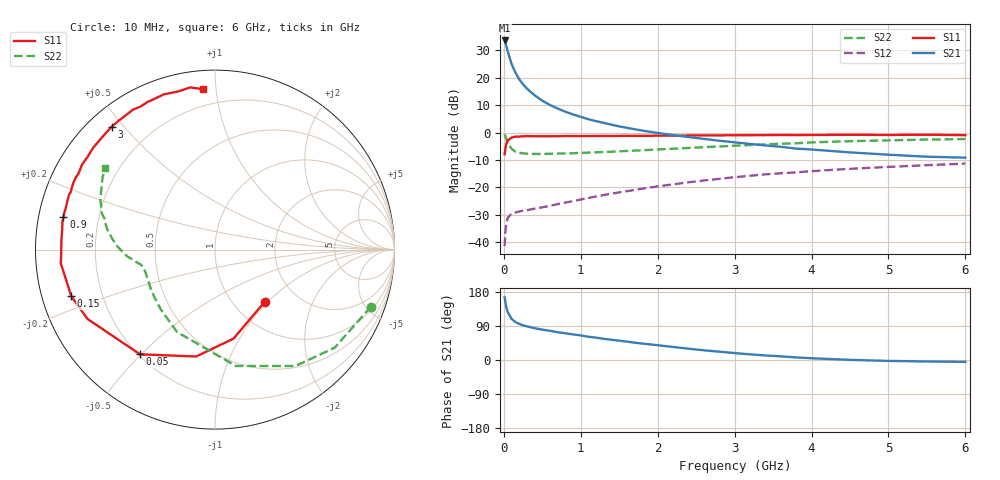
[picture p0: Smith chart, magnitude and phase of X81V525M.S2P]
! SIEMENS Small Signal Semiconductors
! BFP136W
! Si NPN RF Bipolar Junction Transistor in SOT343
! VCE = 1.5 V  IC = 25 mA
! Common Emitter S-Parameters:  September  1994
# GHz  S  MA  R  50
!  f  S11  S21  S12  S22
! GHz  MAG  ANG  MAG  ANG  MAG  ANG  MAG  ANG
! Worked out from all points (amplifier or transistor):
!   40 points, 10 MHz to 6 GHz, reference 50 ohm
!   highest |S21| = 33.6 dB at 10 MHz (marker M1)
!   |S21| within 3 dB of that: start of sweep to 41.63 MHz
!   unconditionally stable (mu >= 1): 768.6 MHz to 2.874 GHz
!   at 200 MHz: K = 0.39, MSG = 24.1 dB, |S12| = -28.8 dB
!   at 1.5 GHz: K = 1.16, MAG = 9.6 dB, |S12| = -21.8 dB
!   at 6 GHz: K = 1.00, MSG = 1.1 dB, |S12| = -11.3 dB
!   S11 on the Smith chart (normalised r, x): 10 MHz: 1.38, -0.96; 50 MHz: 0.21, -0.50; 150 MHz: 0.09, -0.16; 900 MHz: 0.07, +0.10; 3 GHz: 0.07, +0.46; 6 GHz: 0.10, +0.92
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0.01  0.4017 -46.4  47.72 165.4  0.0085 74.6  0.9248 -20.1
0.02  0.5068 -78.3  43.52 152.2  0.0155 63.8  0.8623 -39.3
0.03  0.6048 -100.0  39.22 141.5  0.0213 54.4  0.7888 -55.3
0.05  0.7175 -125.6  30.34 126.3  0.0278 41.0  0.659 -79.8
0.1  0.8089 -151.5  17.9 108.6  0.0334 28.8  0.5053 -114.8
0.15  0.842 -162.1  12.38 100.2  0.0349 25.6  0.4496 -132.3
0.2  0.8457 -167.9  9.362 95.2  0.0364 25.2  0.4282 -142.6
0.25  0.8538 -172.0  7.568 91.5  0.0376 26.1  0.4184 -149.1
0.3  0.8624 -174.8  6.342 88.8  0.0384 27.5  0.4117 -153.6
0.4  0.8565 -179.7  4.777 84.0  0.0411 30.4  0.408 -159.2
0.5  0.8574 177.0  3.809 80.1  0.0434 34.0  0.4078 -162.7
0.6  0.8572 174.8  3.182 77.0  0.0463 37.1  0.4101 -164.8
0.7  0.8595 171.9  2.738 73.3  0.0496 40.1  0.413 -166.2
0.9  0.8636 168.0  2.14 67.5  0.0564 44.2  0.4202 -168.4
1.1  0.8638 163.5  1.749 61.3  0.0643 47.4  0.4308 -169.7
1.6  0.8729 154.4  1.219 48.5  0.0854 51.6  0.462 -172.9
2.2  0.8784 143.9  0.899 34.3  0.114 51.7  0.5067 -177.6
3  0.8946 130.0  0.664 18.3  0.1536 47.3  0.5752 174.1
3.2  0.8965 126.6  0.62 14.9  0.163 45.8  0.5917 171.7
4.5  0.9107 108.2  0.435 0.4  0.2184 34.3  0.6964 156.5
5.5  0.914 98.7  0.363 -3.9  0.2543 26.1  0.7453 147.2
6  0.8962 94.2  0.349 -4.9  0.2719 21.6  0.7625 143.4
